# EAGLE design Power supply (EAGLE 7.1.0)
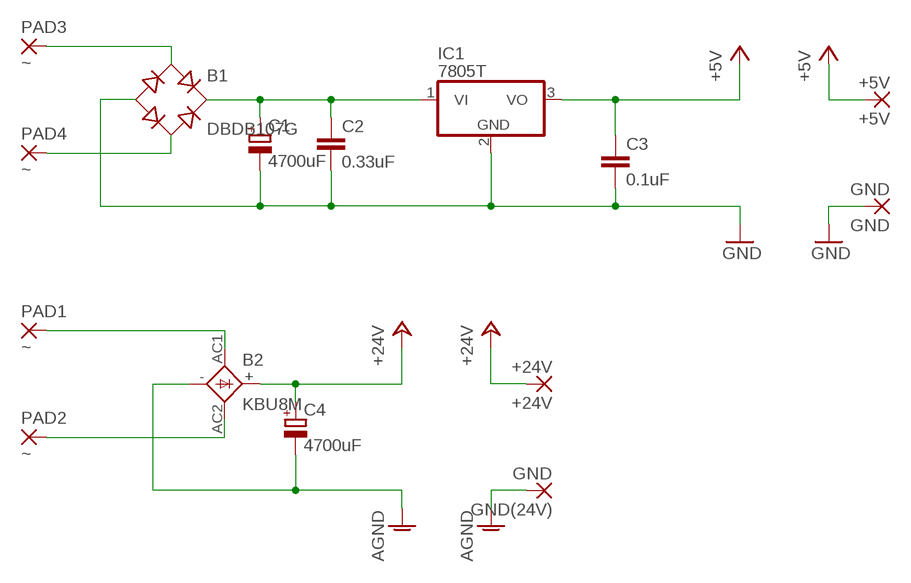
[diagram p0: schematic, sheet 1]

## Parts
+5V  +5V  3,81/1,1  [3,81/1,1]
+24V  +24V  3,81/1,1  [3,81/1,1]
B1  DBDB107G  [DB]
B2  KBU8M  KBU  [KBU]
C1  4700uF  CPOL-EUE5-13  [E5-13]
C2  0.33uF  C-EU050-024X044  [C050-024X044]
C3  0.1uF  C-EU050-024X044  [C050-024X044]
C4  4700uF  CPOL-EUE10-22.5  [EB22,5D]
GND  GND  3,81/1,1  [3,81/1,1]
GND(24V)  GND  3,81/1,1  [3,81/1,1]
IC1  7805T  [TO220H]
PAD1  ~  3,81/1,1  [3,81/1,1]
PAD2  ~  3,81/1,1  [3,81/1,1]
PAD3  ~  3,81/1,1  [3,81/1,1]
PAD4  ~  3,81/1,1  [3,81/1,1]

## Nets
+5V: +5V.1(P) C3.1 IC1.3(VO)
+24V: +24V.1(P) B2.+ C4.+
AGND: B2.- C4.- GND(24V).1(P)
GND: B1.- C1.- C2.2 C3.2 GND.1(P) IC1.2(GND)
N$1: B2.AC1 PAD1.1(P)
N$2: B2.AC2 PAD2.1(P)
N$5: B1.AC1 PAD3.1(P)
N$6: B1.AC2 PAD4.1(P)
N$8: B1.+ C1.+ C2.1 IC1.1(VI)

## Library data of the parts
+5V +24V GND GND(24V) PAD1-PAD4 = wirepad:3,81/1,1: THROUGH-HOLE PAD
B1 = rectifier:DB?*G: Single Phase 1.0 AMP Glass Passivated Bridge Rectifier Taiwan Semiconductor Co.,Ltd. - TSC Source: http://www.taiwansemi.com/TSCbig5/ezcatfiles/cust/img/img/db101g.pdf http://www.ts.com.tw/db/pictures/modules/PDT/PDT060207001/DBLS201G.pdf
B2 = rectifier:KBU: DIOTEC RECTIFIER
C1 C4 = rcl:CPOL-EU: POLARIZED CAPACITOR, European symbol
C2 C3 = rcl:C-EU: CAPACITOR, European symbol
IC1 = linear:78*: Positive VOLTAGE REGULATOR Source: http://cache.national.com/ds/LM/LM78L05.pdf http://www.fairchildsemi.com/ds/LM/LM7805.pdf

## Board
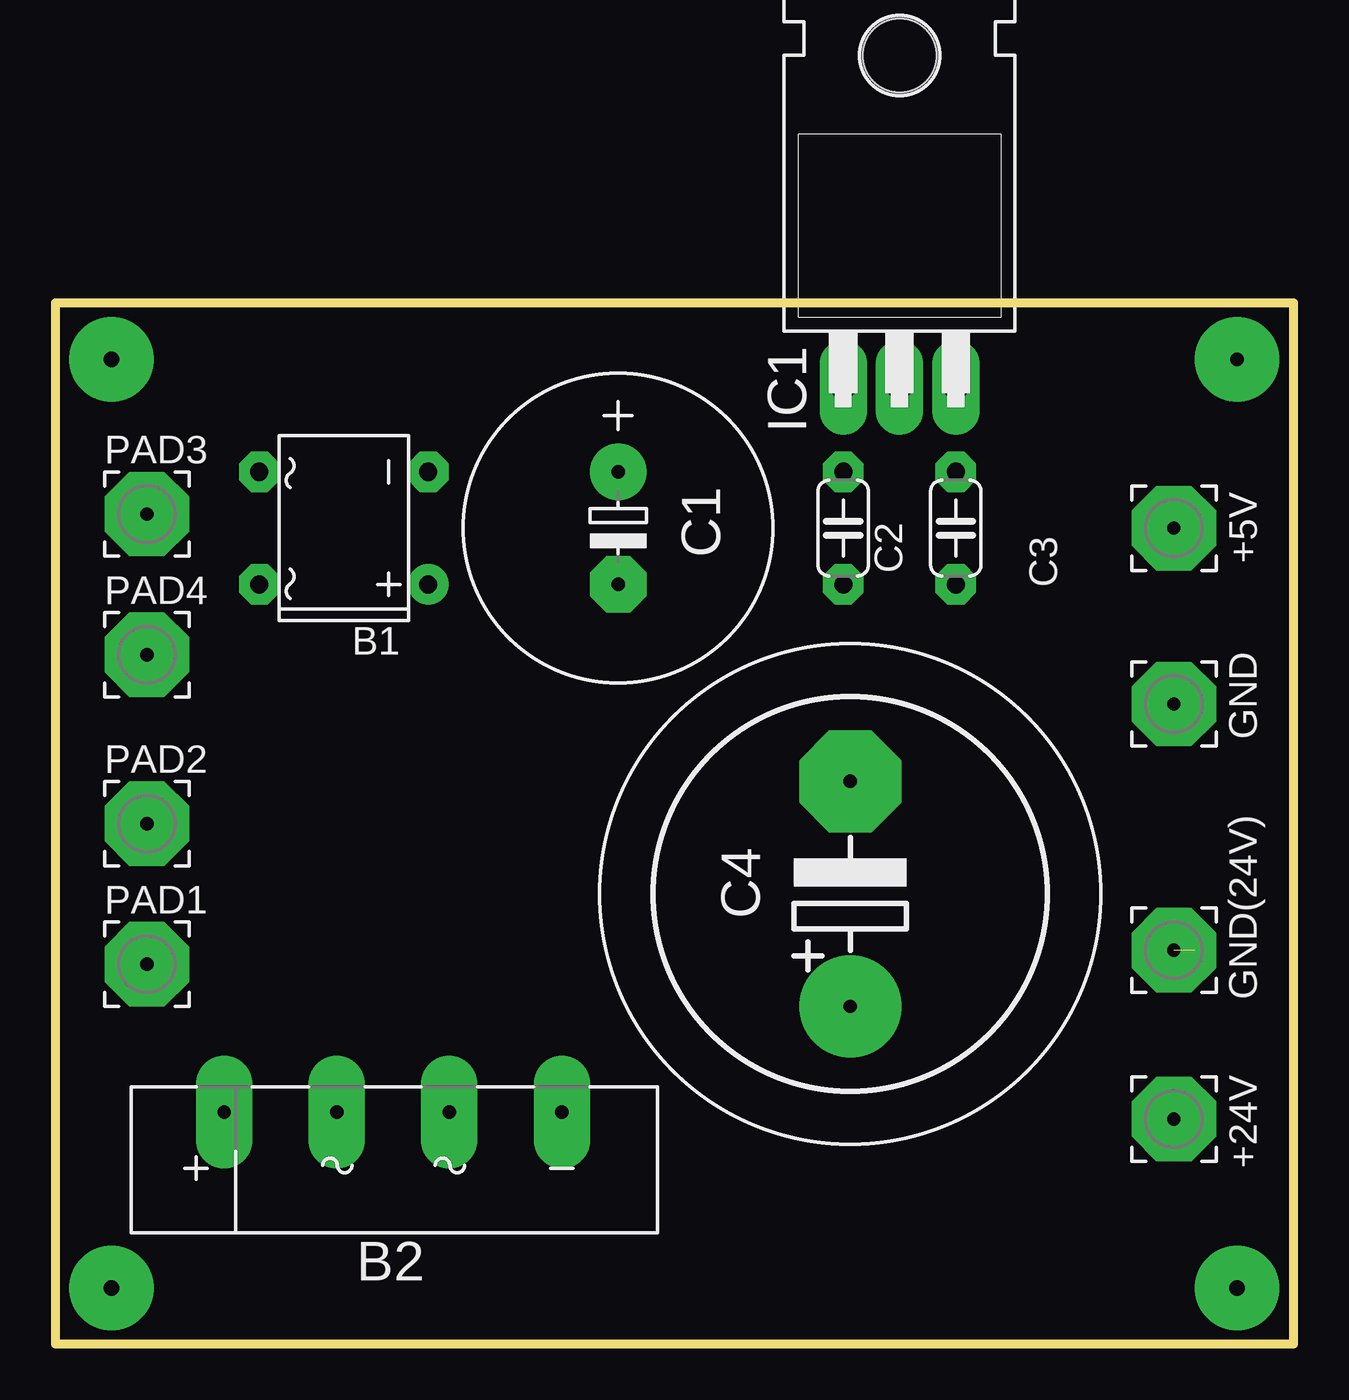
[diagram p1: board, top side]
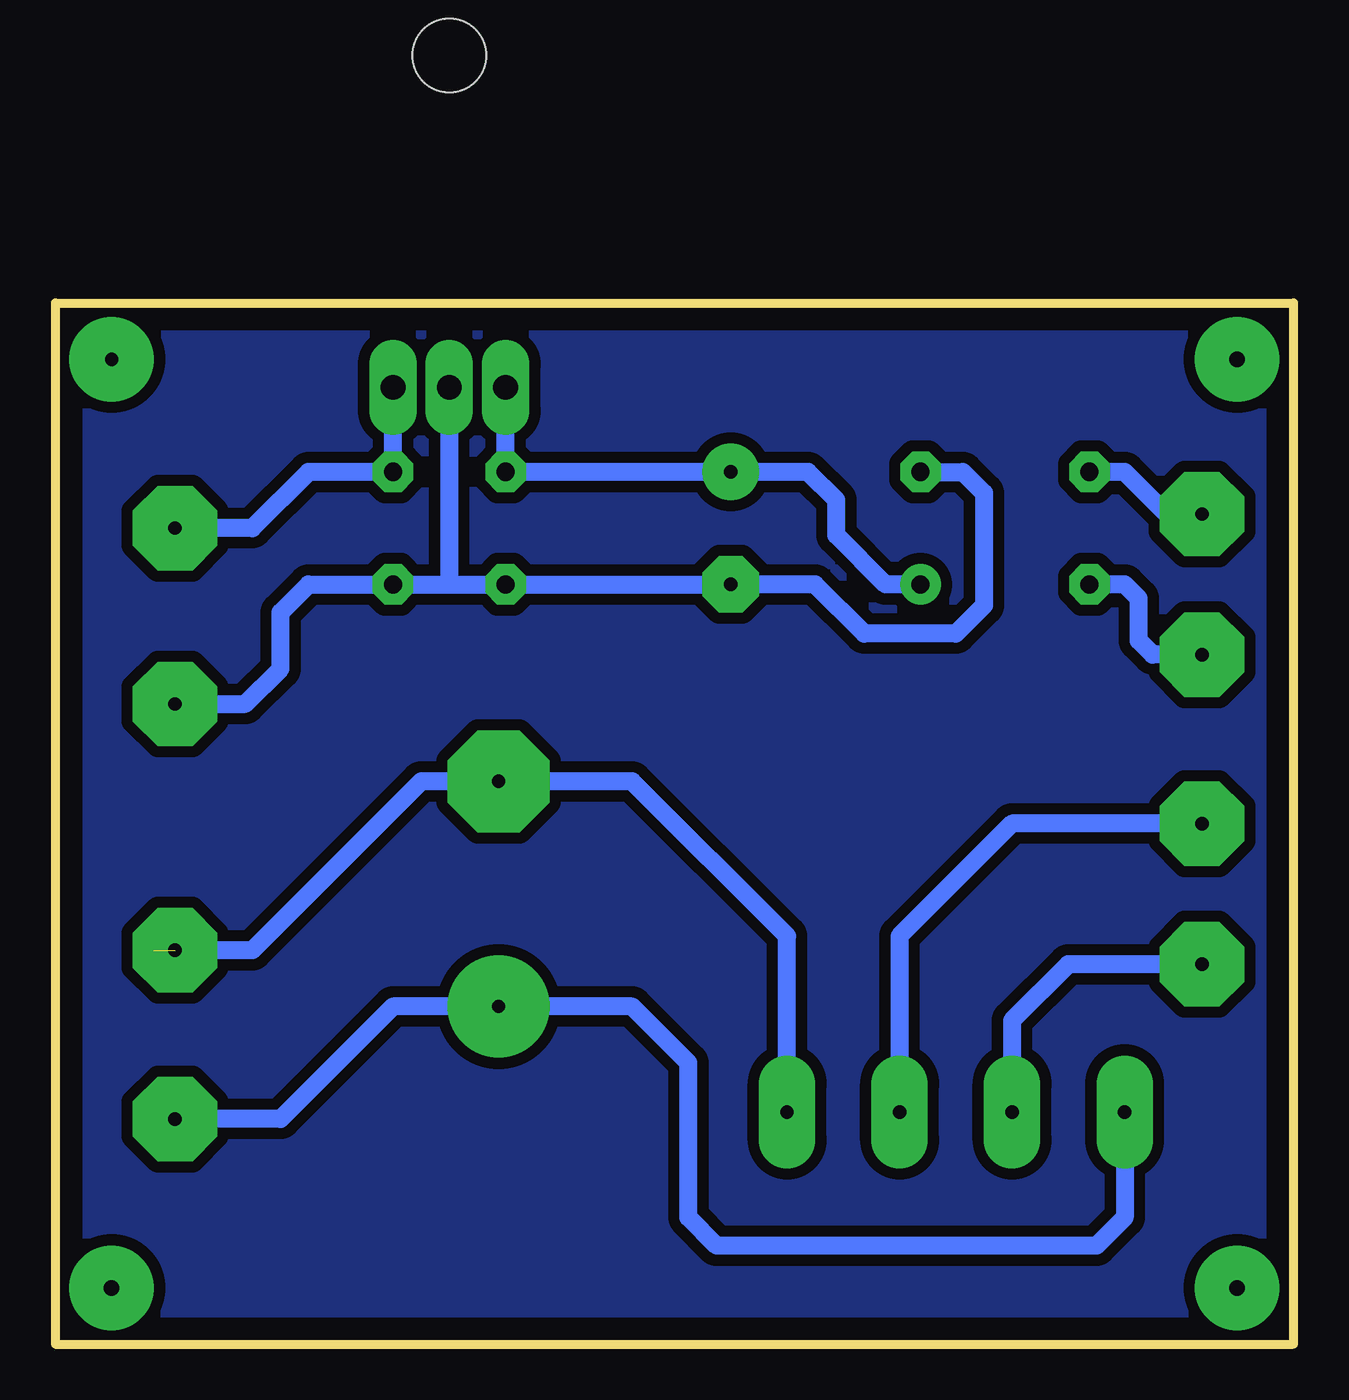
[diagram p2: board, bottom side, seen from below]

Size 55.88 x 46.99 mm. Coordinates in mm from the lower left corner, seen from the top.
Outline: 55.88,46.99 0,46.99 0,0 55.88,0 55.88,46.99
Copper layers (1*16): Top 0.035mm / dielectric 1.5mm / Bottom 0.035mm
Design rules "default *": minimum track width 12mil, minimum drill 20mil, track to track 20mil, track to pad 12mil, pad to pad 12mil, via to via 12mil, smd to smd 12mil, copper to edge 40mil, drill to drill 20mil, minimum pad ring 20mil, minimum via ring 20mil, stop-mask expansion 4mil, vias tented up to drill 0mil, thermal gap 10mil

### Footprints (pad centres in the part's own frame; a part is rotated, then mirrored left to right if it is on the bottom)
3,81/1,1 = drill 0.6 pad 3.81 octagon: 1 0,0
DB = drill 0.813: + -2.54,-3.81 | drill 0.813 octagon: - 2.54,-3.81; AC1 2.54,3.81; AC2 -2.54,3.81
KBU = drill 0.6 pad 2.54 long: + -7.62,2.54; - 7.62,2.54; AC1 -2.54,2.54; AC2 2.54,2.54
E5-13 = drill 0.6 pad 2.54: + -2.54,0 | drill 0.6 pad 2.54 octagon: - 2.54,0
C050-024X044 = drill 0.813 octagon: 1 -2.54,0; 2 2.54,0
EB22,5D = drill 0.6 pad 4.597: + -5.08,0 | drill 0.6 pad 4.597 octagon: - 5.08,0
TO220H = drill 1.118 long: 1 -2.54,-10.16; 2 0,-10.16; 3 2.54,-10.16 | hole 3.302: 0,4.826

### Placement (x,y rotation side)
+5V  50.48,36.83 0 top
+24V  50.48,10.16 0 top
B1  13.02,36.83 90 top
B2  15.24,7.94 0 top
C1  25.4,36.83 270 top
C2  35.56,36.83 270 top
C3  40.64,36.83 270 top
C4  35.88,20.32 90 top
GND  50.48,28.89 0 top
GND(24V)  50.48,17.78 0 top
IC1  38.1,53.34 0 top
PAD1  4.13,17.14 0 top
PAD2  4.13,23.49 0 top
PAD3  4.13,37.46 0 top
PAD4  4.13,31.11 0 top

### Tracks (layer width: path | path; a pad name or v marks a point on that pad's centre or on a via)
+5V
  Bottom 0.813: IC1.3 C3.1 44.45,39.37 46.99,36.83 +5V.1
+24V
  Bottom 0.813: +24V.1 45.72,10.16 40.64,15.24 C4.+ 29.84,15.24 27.3,12.7 27.3,5.71 26.03,4.45 8.89,4.45 7.62,5.71 B2.+
AGND  (1 unrouted)
  Bottom 0.813: 51.43,17.78 46.99,17.78 39.37,25.4 C4.- 29.84,25.4 22.86,18.41 B2.-
GND
  Bottom 0.813: IC1.2 38.1,34.29 | 38.1,34.29 C2.2 C1.- 21.59,34.29 19.37,32.07 15.24,32.07 13.97,33.34 13.97,38.42 14.92,39.37 B1.- | 38.1,34.29 C3.2 44.45,34.29 45.72,33.02 45.72,30.48 47.31,28.89 GND.1
N$1
  Bottom 0.813: PAD1.1 10.16,17.14 12.7,14.61 B2.AC1
N$2
  Bottom 0.813: PAD2.1 12.7,23.49 17.78,18.41 B2.AC2
N$3  (via drill 0.7 pad 3.81)
  other vias: 2.54,44.45
N$4  (via drill 0.6 pad 3.81)
  other vias: 53.34,44.45
N$5
  Bottom 0.813: PAD3.1 5.71,37.46 7.62,39.37 B1.AC1
N$6
  Bottom 0.813: PAD4.1 6.35,31.11 6.98,31.75 6.98,33.66 7.62,34.29 B1.AC2
N$7  (via drill 0.7 pad 3.81)
  other vias: 53.34,2.54
N$8
  Bottom 0.813: IC1.1 C2.1 C1.+ 21.91,39.37 20.64,38.1 20.64,36.51 18.41,34.29 B1.+
N$9  (via drill 0.7 pad 3.81)
  other vias: 2.54,2.54
N$10
  pour Bottom: 0.63,46.35 0.63,0.64 55.24,0.64 55.24,46.35

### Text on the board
tValues: ~ | ~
